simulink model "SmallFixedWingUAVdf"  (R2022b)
settings: Solver=ode4  StartTime=0  StopTime=stoptime  FixedStep=0.001  RelTol=1e-3  EnableMultiTasking=on
PreLoadFcn:
  | asbswarm_vehicledata; % load in workspace variables
PostLoadFcn:
  | open_system([gcs,'/MATLAB Animation Display/MATLAB',10,'Animation']);
InitFcn:
  | InitDatactrl
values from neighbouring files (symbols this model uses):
  env = struct    [InitDatactrl.m]
  F = Fattr + Frep    [APF.m]
  q = ix-1    [bspline_deboor.m]
  SenorSampleTime = 0.01    [InitDatactrl.m]
  sensors = struct    [InitDatactrl.m]
  uav = struct    [InitDatactrl.m]    (also in InitDatactrldf.m)
undefined symbols (not defined in the file or in its folder): Busy, Continuous, DiscIntNeverNeededParam, Dryden, Earth, Light, MIL, Newton, pa28, r, Raphson, sigbuilder_block, Wait, WGS84
libraries: simulink x37, aerolibactuator x10, sharedtransform x6, aerolibatmos2 x4, aerolibasang x4, aerolibwind2 x4, aerolibtransform2 x3, aerolibconvert2 x3, aerolibfltsims x2, shared6dof x2, aerolibnav x2, aerolibanimutils x1
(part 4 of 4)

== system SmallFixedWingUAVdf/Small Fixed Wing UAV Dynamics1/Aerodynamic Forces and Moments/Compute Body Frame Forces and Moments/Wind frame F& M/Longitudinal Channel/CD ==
  CL : Inport
  dE : Inport  Port=2
  dR : Inport  Port=3
  Apolar : Constant  Value=uav.aero.CLmin
  Apolar (A2) : Constant  Value=uav.aero.e
  Apolar (A2)1 : Constant  Value=uav.geometry.AR
  CD0 : Constant  Value=uav.aero.CD0
  CD1 : Constant  Value=uav.aero.CDDe
  CD2 : Constant  Value=uav.aero.CDDr
  Constant : Constant  Value=pi
  Product : Product  Inputs=*/  SaturateOnIntegerOverflow=on
  Product1 : Product  Inputs=***  SaturateOnIntegerOverflow=on
  Product2 : Product  SaturateOnIntegerOverflow=on
  Product4 : Product  SaturateOnIntegerOverflow=on
  Sum1 : Sum  Inputs=++++  SaturateOnIntegerOverflow=on
  Sum2 : Sum  Inputs=|+-  SaturateOnIntegerOverflow=on
  CD : Outport  VectorParamsAs1DForOutWhenUnconnected=off
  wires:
  Sum1/1 -> CD/1
  CL/1 -> Sum2/1
  CD0/1 -> Sum1/1
  Apolar/1 -> Sum2/2
  CD1/1 -> Product4/1
  dE/1 -> Product4/2
  dR/1 -> Product2/2
  CD2/1 -> Product2/1
  Sum2/1 -> Product/1
  Product4/1 -> Sum1/2
  Product2/1 -> Sum1/3
  Product/1 -> Sum1/4
  Apolar (A2)1/1 -> Product1/1
  Apolar (A2)/1 -> Product1/3
  Constant/1 -> Product1/2
  Product1/1 -> Product/2

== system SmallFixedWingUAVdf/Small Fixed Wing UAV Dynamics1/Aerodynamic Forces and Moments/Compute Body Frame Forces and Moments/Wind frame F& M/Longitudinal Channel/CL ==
  alpha : Inport
  alpha_dot : Inport  Port=2
  dE : Inport  Port=3
  dF : Inport  Port=4
  p,q,r : Inport  Port=5
  Airspeed : Inport  Port=6
  CL0 : Constant  Value=uav.aero.CL0
  CLDe : Constant  Value=uav.aero.CLDe
  CLa : Constant  Value=uav.aero.CLa
  CmDe1 : Constant  Value=uav.aero.CLDf
  Lift due to attack rate : Subsystem
  Lift due to pitch rate : Subsystem
  Product1 : Product  SaturateOnIntegerOverflow=on
  Product2 : Product  SaturateOnIntegerOverflow=on
  Product4 : Product  SaturateOnIntegerOverflow=on
  Sum : Sum  Inputs=++++++  SaturateOnIntegerOverflow=on
  CL : Outport  VectorParamsAs1DForOutWhenUnconnected=off
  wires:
  CL0/1 -> Sum/1
  Airspeed/1 -> Lift due to attack rate/1(Airspeed), Lift due to pitch rate/2(Airspeed)
  p,q,r/1 -> Lift due to pitch rate/1(p,q,r)
  Lift due to pitch rate/1(CLq) -> Sum/5
  Product2/1 -> Sum/4
  Product1/1 -> Sum/3
  CmDe1/1 -> Product2/1
  dF/1 -> Product2/2
  Sum/1 -> CL/1
  dE/1 -> Product1/2
  CLDe/1 -> Product1/1
  alpha/1 -> Product4/2
  CLa/1 -> Product4/1
  alpha_dot/1 -> Lift due to attack rate/2(alpha_dot)
  Lift due to attack rate/1(CLadot) -> Sum/6
  Product4/1 -> Sum/2

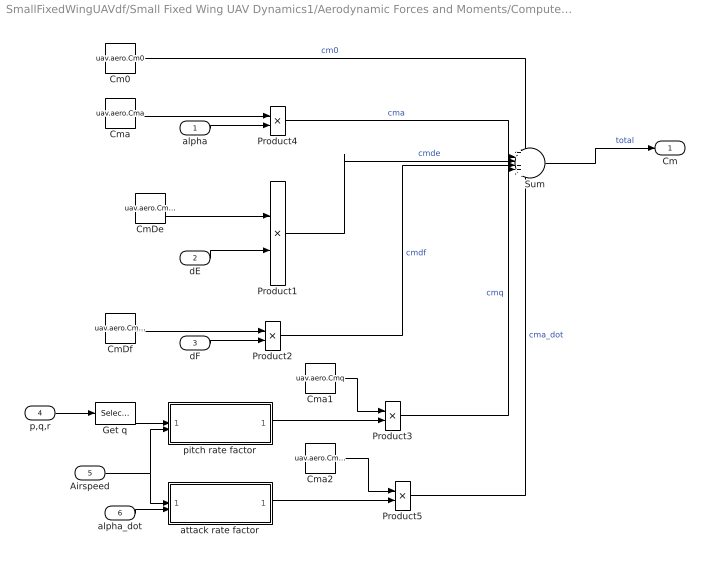
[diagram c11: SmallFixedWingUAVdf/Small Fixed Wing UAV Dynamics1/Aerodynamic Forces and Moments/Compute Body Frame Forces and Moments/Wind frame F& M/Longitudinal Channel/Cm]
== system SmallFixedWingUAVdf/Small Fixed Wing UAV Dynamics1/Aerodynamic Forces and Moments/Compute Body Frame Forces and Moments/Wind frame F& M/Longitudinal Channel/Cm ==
  alpha : Inport
  dE : Inport  Port=2
  dF : Inport  Port=3
  p,q,r : Inport  Port=4
  Airspeed : Inport  Port=5
  alpha_dot : Inport  Port=6
  Cm0 : Constant  Value=uav.aero.Cm0
  CmDe : Constant  Value=uav.aero.CmDe
  CmDf : Constant  Value=uav.aero.CmDf
  Cma : Constant  Value=uav.aero.Cma
  Cma1 : Constant  Value=uav.aero.Cmq
  Cma2 : Constant  Value=uav.aero.Cma_dot
  Get q : Selector  InputPortWidth=3  IndexOptions=Index vector (dialog)  Indices=2  OutputSizes=[(-2)]
  Product1 : Product  Inputs=**  SaturateOnIntegerOverflow=on
  Product{2..5} (4 alike) : Product  SaturateOnIntegerOverflow=on
  Sum : Sum  Inputs=++++++  SaturateOnIntegerOverflow=on
  attack rate factor : Subsystem
  pitch rate factor : Subsystem
  Cm : Outport  VectorParamsAs1DForOutWhenUnconnected=off
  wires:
  Product3/1 -> Sum/5  "cmq"
  p,q,r/1 -> Get q/1
  Product1/1 -> Sum/3  "cmde"
  Product4/1 -> Sum/2  "cma"
  Sum/1 -> Cm/1  "total"
  dE/1 -> Product1/2
  CmDe/1 -> Product1/1
  alpha/1 -> Product4/2
  Cma/1 -> Product4/1
  dF/1 -> Product2/2
  CmDf/1 -> Product2/1
  Product2/1 -> Sum/4  "cmdf"
  Cm0/1 -> Sum/1  "cm0"
  alpha_dot/1 -> attack rate factor/2(alpha_dot)
  Get q/1 -> pitch rate factor/1(q)
  Airspeed/1 -> attack rate factor/1(Airspeed), pitch rate factor/2(Airspeed)
  Cma1/1 -> Product3/1
  pitch rate factor/1(Pitch Rate Fac) -> Product3/2
  attack rate factor/1(Pitch Rate Fac) -> Product5/2
  Cma2/1 -> Product5/1
  Product5/1 -> Sum/6  "cma_dot"

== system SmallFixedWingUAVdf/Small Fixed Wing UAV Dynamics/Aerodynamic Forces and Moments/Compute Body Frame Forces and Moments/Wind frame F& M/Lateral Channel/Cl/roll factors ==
  p,q,r : Inport
  Airspeed : Inport  Port=2
  Constant : Constant  Value=uav.aero.Clp
  Constant1 : Constant  Value=uav.aero.Clr
  Get p : Selector  InputPortWidth=3  IndexOptions=Index vector (dialog)  Indices=1  OutputSizes=[(-2)]
  Get r : Selector  InputPortWidth=3  IndexOptions=Index vector (dialog)  Indices=3  OutputSizes=[(-2)]
  Product : Product  SaturateOnIntegerOverflow=on
  Product1 : Product  SaturateOnIntegerOverflow=on
  roll rate fact : Subsystem
  yaw rate fact1 : Subsystem
  Clp : Outport  VectorParamsAs1DForOutWhenUnconnected=off
  Clr : Outport  Port=2  VectorParamsAs1DForOutWhenUnconnected=off
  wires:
  Get r/1 -> yaw rate fact1/1(r)
  p,q,r/1 -> Get r/1, Get p/1
  Get p/1 -> roll rate fact/1(p)
  Airspeed/1 -> yaw rate fact1/2(Airspeed), roll rate fact/2(Airspeed)
  yaw rate fact1/1(Yaw Rate Fac) -> Product1/2
  Constant1/1 -> Product1/1
  roll rate fact/1(Roll Rate Fac) -> Product/2
  Constant/1 -> Product/1
  Product1/1 -> Clr/1
  Product/1 -> Clp/1

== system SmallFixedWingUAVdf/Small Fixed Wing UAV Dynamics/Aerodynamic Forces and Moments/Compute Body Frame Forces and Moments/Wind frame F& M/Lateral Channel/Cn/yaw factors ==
  p,q,r : Inport
  Airspeed : Inport  Port=2
  Constant : Constant  Value=uav.aero.Cnp
  Constant1 : Constant  Value=uav.aero.Cnr
  Get p : Selector  InputPortWidth=3  IndexOptions=Index vector (dialog)  Indices=1  OutputSizes=[(-2)]
  Get r : Selector  InputPortWidth=3  IndexOptions=Index vector (dialog)  Indices=3  OutputSizes=[(-2)]
  Product : Product  SaturateOnIntegerOverflow=on
  Product1 : Product  SaturateOnIntegerOverflow=on
  roll rate fact : Subsystem
  yaw rate fact : Subsystem
  Cnp : Outport  VectorParamsAs1DForOutWhenUnconnected=off
  Cnr : Outport  Port=2  VectorParamsAs1DForOutWhenUnconnected=off
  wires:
  Airspeed/1 -> yaw rate fact/2(Airspeed), roll rate fact/2(Airspeed)
  Get r/1 -> yaw rate fact/1(r)
  p,q,r/1 -> Get r/1, Get p/1
  Get p/1 -> roll rate fact/1(p)
  roll rate fact/1(Roll Rate Fac) -> Product/2
  Constant/1 -> Product/1
  yaw rate fact/1(Yaw Rate Fac) -> Product1/2
  Constant1/1 -> Product1/1
  Product1/1 -> Cnr/1
  Product/1 -> Cnp/1

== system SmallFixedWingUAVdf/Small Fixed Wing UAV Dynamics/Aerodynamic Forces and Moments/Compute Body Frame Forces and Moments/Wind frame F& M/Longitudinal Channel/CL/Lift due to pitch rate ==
  p,q,r : Inport
  Airspeed : Inport  Port=2
  Constant : Constant  Value=uav.aero.CLq
  Get q : Selector  InputPortWidth=3  IndexOptions=Index vector (dialog)  Indices=2  OutputSizes=[(-2)]
  Product : Product  SaturateOnIntegerOverflow=on
  pitch rate factor : Subsystem
  CLq : Outport  VectorParamsAs1DForOutWhenUnconnected=off
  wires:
  Airspeed/1 -> pitch rate factor/2(Airspeed)
  Get q/1 -> pitch rate factor/1(q)
  p,q,r/1 -> Get q/1
  Product/1 -> CLq/1
  pitch rate factor/1(Pitch Rate Fac) -> Product/2
  Constant/1 -> Product/1

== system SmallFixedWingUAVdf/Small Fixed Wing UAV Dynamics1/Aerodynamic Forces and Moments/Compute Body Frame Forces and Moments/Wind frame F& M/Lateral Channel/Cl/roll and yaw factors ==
  p,q,r : Inport
  Airspeed : Inport  Port=2
  Constant : Constant  Value=uav.aero.Clp
  Constant1 : Constant  Value=uav.aero.Clr
  Get p : Selector  InputPortWidth=3  IndexOptions=Index vector (dialog)  Indices=1  OutputSizes=[(-2)]
  Get r : Selector  InputPortWidth=3  IndexOptions=Index vector (dialog)  Indices=3  OutputSizes=[(-2)]
  Product : Product  SaturateOnIntegerOverflow=on
  Product1 : Product  SaturateOnIntegerOverflow=on
  roll rate fact : Subsystem
  yaw rate fact : Subsystem
  Clp : Outport  VectorParamsAs1DForOutWhenUnconnected=off
  Clr : Outport  Port=2  VectorParamsAs1DForOutWhenUnconnected=off
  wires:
  Get r/1 -> yaw rate fact/1(r)
  p,q,r/1 -> Get r/1, Get p/1
  Get p/1 -> roll rate fact/1(p)
  Airspeed/1 -> yaw rate fact/2(Airspeed), roll rate fact/2(Airspeed)
  yaw rate fact/1(Yaw Rate Fac) -> Product1/2
  Constant1/1 -> Product1/1
  roll rate fact/1(Roll Rate Fac) -> Product/2
  Constant/1 -> Product/1
  Product1/1 -> Clr/1
  Product/1 -> Clp/1

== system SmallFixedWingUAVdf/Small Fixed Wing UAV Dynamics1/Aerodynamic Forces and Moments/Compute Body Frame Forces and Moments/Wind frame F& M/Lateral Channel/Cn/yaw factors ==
  p,q,r : Inport
  Airspeed : Inport  Port=2
  Constant : Constant  Value=uav.aero.Cnp
  Constant1 : Constant  Value=uav.aero.Cnr
  Get p : Selector  InputPortWidth=3  IndexOptions=Index vector (dialog)  Indices=1  OutputSizes=[(-2)]
  Get r : Selector  InputPortWidth=3  IndexOptions=Index vector (dialog)  Indices=3  OutputSizes=[(-2)]
  Product : Product  SaturateOnIntegerOverflow=on
  Product1 : Product  SaturateOnIntegerOverflow=on
  roll rate fact : Subsystem
  yaw rate fact : Subsystem
  Cnp : Outport  VectorParamsAs1DForOutWhenUnconnected=off
  Cnr : Outport  Port=2  VectorParamsAs1DForOutWhenUnconnected=off
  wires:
  Airspeed/1 -> yaw rate fact/2(Airspeed), roll rate fact/2(Airspeed)
  Get r/1 -> yaw rate fact/1(r)
  p,q,r/1 -> Get r/1, Get p/1
  Get p/1 -> roll rate fact/1(p)
  roll rate fact/1(Roll Rate Fac) -> Product/2
  Constant/1 -> Product/1
  yaw rate fact/1(Yaw Rate Fac) -> Product1/2
  Constant1/1 -> Product1/1
  Product1/1 -> Cnr/1
  Product/1 -> Cnp/1

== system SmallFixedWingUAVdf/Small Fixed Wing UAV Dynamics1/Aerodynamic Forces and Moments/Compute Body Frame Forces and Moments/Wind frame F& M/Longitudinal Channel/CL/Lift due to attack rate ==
  Airspeed : Inport
  alpha_dot : Inport  Port=2
  CLa_dot : Constant  Value=uav.aero.CLa_dot
  Product : Product  SaturateOnIntegerOverflow=on
  attack rate factor : Subsystem
  CLadot : Outport  VectorParamsAs1DForOutWhenUnconnected=off
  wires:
  Airspeed/1 -> attack rate factor/1(Airspeed)
  alpha_dot/1 -> attack rate factor/2(alpha_dot)
  Product/1 -> CLadot/1
  attack rate factor/1(Pitch Rate Fac) -> Product/2
  CLa_dot/1 -> Product/1

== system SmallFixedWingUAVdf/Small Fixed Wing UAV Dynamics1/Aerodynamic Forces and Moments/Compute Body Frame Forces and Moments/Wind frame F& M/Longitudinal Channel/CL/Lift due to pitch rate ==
  p,q,r : Inport
  Airspeed : Inport  Port=2
  Constant : Constant  Value=uav.aero.CLq
  Get q : Selector  InputPortWidth=3  IndexOptions=Index vector (dialog)  Indices=2  OutputSizes=[(-2)]
  Product : Product  SaturateOnIntegerOverflow=on
  pitch rate factor : Subsystem
  CLq : Outport  VectorParamsAs1DForOutWhenUnconnected=off
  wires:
  Airspeed/1 -> pitch rate factor/2(Airspeed)
  Get q/1 -> pitch rate factor/1(q)
  p,q,r/1 -> Get q/1
  Product/1 -> CLq/1
  pitch rate factor/1(Pitch Rate Fac) -> Product/2
  Constant/1 -> Product/1

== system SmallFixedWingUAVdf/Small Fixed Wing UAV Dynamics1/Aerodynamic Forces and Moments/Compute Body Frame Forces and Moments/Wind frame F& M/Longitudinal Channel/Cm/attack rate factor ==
  Airspeed : Inport
  alpha_dot : Inport  Port=2
  Cmq2 : Constant  Value=uav.geometry.chord
  Cmq3 : Constant  Value=.5
  Product : Product  Inputs=***/  SaturateOnIntegerOverflow=on
  Saturation : Saturate  UpperLimit=inf  LowerLimit=0.1
  Pitch Rate Fac : Outport  VectorParamsAs1DForOutWhenUnconnected=off
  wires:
  Saturation/1 -> Product/4
  Cmq2/1 -> Product/2
  Airspeed/1 -> Saturation/1
  Product/1 -> Pitch Rate Fac/1
  alpha_dot/1 -> Product/1
  Cmq3/1 -> Product/3

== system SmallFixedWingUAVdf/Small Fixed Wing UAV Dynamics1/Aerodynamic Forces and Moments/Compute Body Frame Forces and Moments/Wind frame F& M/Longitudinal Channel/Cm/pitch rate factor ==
  q : Inport
  Airspeed : Inport  Port=2
  Cmq2 : Constant  Value=uav.geometry.chord
  Cmq3 : Constant  Value=.5
  Product : Product  Inputs=***/  SaturateOnIntegerOverflow=on
  Saturation : Saturate  UpperLimit=inf  LowerLimit=0.1
  Pitch Rate Fac : Outport  VectorParamsAs1DForOutWhenUnconnected=off
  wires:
  Saturation/1 -> Product/4
  Cmq2/1 -> Product/2
  Airspeed/1 -> Saturation/1
  q/1 -> Product/1
  Product/1 -> Pitch Rate Fac/1
  Cmq3/1 -> Product/3

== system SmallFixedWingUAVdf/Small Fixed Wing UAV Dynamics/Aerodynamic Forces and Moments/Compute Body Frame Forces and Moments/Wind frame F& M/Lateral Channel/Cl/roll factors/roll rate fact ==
  p : Inport
  Airspeed : Inport  Port=2
  Cmq1 : Constant  Value=.5
  Cmq2 : Constant  Value=uav.geometry.span
  Product : Product  Inputs=***/  SaturateOnIntegerOverflow=on
  Saturation : Saturate  UpperLimit=inf  LowerLimit=0.1
  Roll Rate Fac : Outport  VectorParamsAs1DForOutWhenUnconnected=off
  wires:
  Saturation/1 -> Product/4
  Airspeed/1 -> Saturation/1
  Cmq2/1 -> Product/3
  Cmq1/1 -> Product/2
  p/1 -> Product/1
  Product/1 -> Roll Rate Fac/1

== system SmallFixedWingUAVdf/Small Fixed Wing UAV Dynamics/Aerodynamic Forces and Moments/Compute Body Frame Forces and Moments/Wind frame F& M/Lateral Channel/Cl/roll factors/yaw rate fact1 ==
  r : Inport
  Airspeed : Inport  Port=2
  Cmq3 : Constant  Value=.5
  Cmq4 : Constant  Value=uav.geometry.span
  Product1 : Product  Inputs=***/  SaturateOnIntegerOverflow=on
  Saturation : Saturate  UpperLimit=inf  LowerLimit=0.1
  Yaw Rate Fac : Outport  VectorParamsAs1DForOutWhenUnconnected=off
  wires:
  Saturation/1 -> Product1/4
  Airspeed/1 -> Saturation/1
  Cmq4/1 -> Product1/3
  Cmq3/1 -> Product1/2
  r/1 -> Product1/1
  Product1/1 -> Yaw Rate Fac/1

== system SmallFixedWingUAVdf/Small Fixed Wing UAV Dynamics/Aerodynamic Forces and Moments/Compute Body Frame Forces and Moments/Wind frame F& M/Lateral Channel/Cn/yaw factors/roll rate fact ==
  p : Inport
  Airspeed : Inport  Port=2
  Cmq1 : Constant  Value=.5
  Cmq2 : Constant  Value=uav.geometry.span
  Product : Product  Inputs=***/  SaturateOnIntegerOverflow=on
  Saturation : Saturate  UpperLimit=inf  LowerLimit=0.1
  Roll Rate Fac : Outport  VectorParamsAs1DForOutWhenUnconnected=off
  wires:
  Saturation/1 -> Product/4
  Airspeed/1 -> Saturation/1
  Cmq2/1 -> Product/3
  Cmq1/1 -> Product/2
  p/1 -> Product/1
  Product/1 -> Roll Rate Fac/1

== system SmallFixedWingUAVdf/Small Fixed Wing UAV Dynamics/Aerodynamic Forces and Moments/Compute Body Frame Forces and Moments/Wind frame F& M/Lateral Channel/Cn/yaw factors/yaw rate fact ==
  r : Inport
  Airspeed : Inport  Port=2
  Cmq3 : Constant  Value=.5
  Cmq4 : Constant  Value=uav.geometry.span
  Product1 : Product  Inputs=***/  SaturateOnIntegerOverflow=on
  Saturation : Saturate  UpperLimit=inf  LowerLimit=0.1
  Yaw Rate Fac : Outport  VectorParamsAs1DForOutWhenUnconnected=off
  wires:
  Product1/1 -> Yaw Rate Fac/1
  r/1 -> Product1/1
  Cmq3/1 -> Product1/2
  Cmq4/1 -> Product1/3
  Airspeed/1 -> Saturation/1
  Saturation/1 -> Product1/4

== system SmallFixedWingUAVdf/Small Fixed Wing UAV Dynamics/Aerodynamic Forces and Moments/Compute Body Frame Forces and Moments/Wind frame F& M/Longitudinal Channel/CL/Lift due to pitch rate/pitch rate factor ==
  q : Inport
  Airspeed : Inport  Port=2
  Cmq2 : Constant  Value=uav.geometry.chord
  Product : Product  Inputs=**/  SaturateOnIntegerOverflow=on
  Saturation : Saturate  UpperLimit=inf  LowerLimit=0.1
  Pitch Rate Fac : Outport  VectorParamsAs1DForOutWhenUnconnected=off
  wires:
  Saturation/1 -> Product/3
  Cmq2/1 -> Product/2
  Airspeed/1 -> Saturation/1
  q/1 -> Product/1
  Product/1 -> Pitch Rate Fac/1

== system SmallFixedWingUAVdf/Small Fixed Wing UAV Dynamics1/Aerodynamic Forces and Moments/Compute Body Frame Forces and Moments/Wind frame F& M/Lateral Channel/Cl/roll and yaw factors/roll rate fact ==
  p : Inport
  Airspeed : Inport  Port=2
  Cmq1 : Constant  Value=.5
  Cmq2 : Constant  Value=uav.geometry.span
  Product : Product  Inputs=***/  SaturateOnIntegerOverflow=on
  Saturation : Saturate  UpperLimit=inf  LowerLimit=0.1
  Roll Rate Fac : Outport  VectorParamsAs1DForOutWhenUnconnected=off
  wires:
  Saturation/1 -> Product/4
  Airspeed/1 -> Saturation/1
  Cmq2/1 -> Product/3
  Cmq1/1 -> Product/2
  p/1 -> Product/1
  Product/1 -> Roll Rate Fac/1

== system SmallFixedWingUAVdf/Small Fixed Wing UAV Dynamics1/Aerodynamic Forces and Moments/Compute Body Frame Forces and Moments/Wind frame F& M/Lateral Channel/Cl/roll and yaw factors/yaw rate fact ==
  r : Inport
  Airspeed : Inport  Port=2
  Cmq3 : Constant  Value=.5
  Cmq4 : Constant  Value=uav.geometry.span
  Product1 : Product  Inputs=***/  SaturateOnIntegerOverflow=on
  Saturation : Saturate  UpperLimit=inf  LowerLimit=0.1
  Yaw Rate Fac : Outport  VectorParamsAs1DForOutWhenUnconnected=off
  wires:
  Product1/1 -> Yaw Rate Fac/1
  r/1 -> Product1/1
  Cmq3/1 -> Product1/2
  Cmq4/1 -> Product1/3
  Airspeed/1 -> Saturation/1
  Saturation/1 -> Product1/4

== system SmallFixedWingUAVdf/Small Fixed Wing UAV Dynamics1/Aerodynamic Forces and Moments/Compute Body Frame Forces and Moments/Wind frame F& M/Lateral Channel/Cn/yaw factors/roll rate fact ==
  p : Inport
  Airspeed : Inport  Port=2
  Cmq1 : Constant  Value=.5
  Cmq2 : Constant  Value=uav.geometry.span
  Product : Product  Inputs=***/  SaturateOnIntegerOverflow=on
  Saturation : Saturate  UpperLimit=inf  LowerLimit=0.1
  Roll Rate Fac : Outport  VectorParamsAs1DForOutWhenUnconnected=off
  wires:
  Saturation/1 -> Product/4
  Airspeed/1 -> Saturation/1
  Cmq2/1 -> Product/3
  Cmq1/1 -> Product/2
  p/1 -> Product/1
  Product/1 -> Roll Rate Fac/1

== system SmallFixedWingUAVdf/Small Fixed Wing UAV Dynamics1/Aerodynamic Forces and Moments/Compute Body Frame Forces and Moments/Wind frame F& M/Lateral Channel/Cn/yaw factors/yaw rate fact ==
  r : Inport
  Airspeed : Inport  Port=2
  Cmq3 : Constant  Value=.5
  Cmq4 : Constant  Value=uav.geometry.span
  Product1 : Product  Inputs=***/  SaturateOnIntegerOverflow=on
  Saturation : Saturate  UpperLimit=inf  LowerLimit=0.1
  Yaw Rate Fac : Outport  VectorParamsAs1DForOutWhenUnconnected=off
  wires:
  Product1/1 -> Yaw Rate Fac/1
  r/1 -> Product1/1
  Cmq3/1 -> Product1/2
  Cmq4/1 -> Product1/3
  Airspeed/1 -> Saturation/1
  Saturation/1 -> Product1/4

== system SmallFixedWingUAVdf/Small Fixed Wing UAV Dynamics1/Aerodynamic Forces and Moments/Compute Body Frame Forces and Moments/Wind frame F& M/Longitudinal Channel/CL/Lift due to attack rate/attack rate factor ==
  Airspeed : Inport
  alpha_dot : Inport  Port=2
  Cmq2 : Constant  Value=uav.geometry.chord
  Product : Product  Inputs=**/  SaturateOnIntegerOverflow=on
  Saturation : Saturate  UpperLimit=inf  LowerLimit=0.1
  Pitch Rate Fac : Outport  VectorParamsAs1DForOutWhenUnconnected=off
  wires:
  Saturation/1 -> Product/3
  Cmq2/1 -> Product/2
  Airspeed/1 -> Saturation/1
  Product/1 -> Pitch Rate Fac/1
  alpha_dot/1 -> Product/1

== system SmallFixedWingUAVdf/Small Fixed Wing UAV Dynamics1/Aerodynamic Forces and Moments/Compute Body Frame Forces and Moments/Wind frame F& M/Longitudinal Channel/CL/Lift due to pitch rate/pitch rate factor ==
  q : Inport
  Airspeed : Inport  Port=2
  Cmq2 : Constant  Value=uav.geometry.chord
  Product : Product  Inputs=**/  SaturateOnIntegerOverflow=on
  Saturation : Saturate  UpperLimit=inf  LowerLimit=0.1
  Pitch Rate Fac : Outport  VectorParamsAs1DForOutWhenUnconnected=off
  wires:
  Saturation/1 -> Product/3
  Cmq2/1 -> Product/2
  Airspeed/1 -> Saturation/1
  q/1 -> Product/1
  Product/1 -> Pitch Rate Fac/1

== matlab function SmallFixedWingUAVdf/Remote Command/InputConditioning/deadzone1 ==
function y = fcn(u)
%Function description:
%  Control the range of the remote control input from RCMin to RCMax, and set
%  a dead zone with a dead zone size of ±deadZone,the output y is
%  normalized to 0~1.You can get the RC calibration parameters in QGC.
RCMin = 1100;
RCMax = 1900;
RCMid = (RCMin + RCMax)/2;
deadZoneRate = 0.05;
deadZone = deadZoneRate*(RCMax - RCMin);
k = 1/(RCMax - RCMid - deadZone);
%Limiting
if(u < RCMin)
    u = RCMin;
elseif(u > RCMax)
    u = RCMax;
end
%dead zone and normalize
 if(u > RCMid + deadZone)
    y = (u-RCMid - deadZone)*k;
 elseif(u < RCMid - deadZone)
     y = (u - RCMid + deadZone)*k;
 else
     y = 0;
 end

 end

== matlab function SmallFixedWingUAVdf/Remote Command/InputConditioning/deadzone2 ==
function y = fcn(u)
%Function description:
%  Control the range of the remote control input from RCMin to RCMax, and set
%  a dead zone with a dead zone size of ±deadZone,the output y is
%  normalized to 0~1.You can get the RC calibration parameters in QGC.
RCMin = 1100;
RCMax = 1900;
RCMid = (RCMin + RCMax)/2;
deadZoneRate = 0.05;
deadZone = deadZoneRate*(RCMax - RCMin);
k = 1/(RCMax - RCMid - deadZone);
%Limiting
if(u < RCMin)
    u = RCMin;
elseif(u > RCMax)
    u = RCMax;
end
%dead zone and normalize
 if(u > RCMid + deadZone)
    y = (u-RCMid - deadZone)*k;
 elseif(u < RCMid - deadZone)
     y = (u - RCMid + deadZone)*k;
 else
     y = 0;
 end

 end

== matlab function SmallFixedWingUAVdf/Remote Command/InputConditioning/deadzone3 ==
function y = fcn(u)
%Function description:
%  Control the range of the remote control input from RCMin to RCMax, and set
%  a dead zone with a dead zone size of ±deadZone,the output y is
%  normalized to 0~1.You can get the RC calibration parameters in QGC.
RCMin = 1100;
RCMax = 1900;
RCMid = (RCMin + RCMax)/2;
deadZoneRate = 0.05;
deadZone = deadZoneRate*(RCMax - RCMin);
k = 1/(RCMax - RCMid - deadZone);
%Limiting
if(u < RCMin)
    u = RCMin;
elseif(u > RCMax)
    u = RCMax;
end
%dead zone and normalize
 if(u > RCMid + deadZone)
    y = (u-RCMid - deadZone)*k;
 elseif(u < RCMid - deadZone)
     y = (u - RCMid + deadZone)*k;
 else
     y = 0;
 end

 end

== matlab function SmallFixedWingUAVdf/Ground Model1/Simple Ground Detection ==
function ifGround = Ground(Xe3)
if Xe3>-(1e-3)
    ifGround = 1;
else
    ifGround = 0;
end

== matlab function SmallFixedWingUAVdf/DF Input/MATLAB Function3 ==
function [av1,Hz,yaw,roll] = DF(xd,dxd,ddxd,x,dx,g)
    
%     x1 = (xd-x)/norm(xd-x);

    r1 = (dxd)/norm(dxd);
    
    av1 =  r1'*(1*ddxd-[0;0;g]+3*(dxd-dx)+0.1*(xd-x));

    an = (eye(3)-r1*r1')*(ddxd-[0;0;g]);

    av3 = -(norm(an));
    
    Hz = xd(3);

    r3 = an/av3;

    r2 = cross(r3,r1);

    yaw = atan2(r1(2),r1(1));
    
    roll = atan2(r2(3),r3(3));

    if isnan(av1)
        av1=0;
    end
    if isnan(Hz)
        Hz=0;
    end
    if isnan(yaw)
        yaw=0;
    end

end

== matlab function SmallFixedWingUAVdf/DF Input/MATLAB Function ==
function roll = fcn(yaw,yawdes,g,V,rolldes)
%     roll = yawrate*g*V;
    if yaw>pi
        yaw = yaw-2*pi;
    end
    yawrate1 = 0.7*(yawdes-yaw);
    roll = atan2(V.*(yawrate1),g);
end

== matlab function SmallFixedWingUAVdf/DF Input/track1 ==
function [Xd,Vd,Ad,Jd] = fcn(x,y,dx,dy,ddx,ddy,dddx,dddy)
    Xd = [x,-y,100]';
    Vd = [dx,-dy,0]';
    Ad = [ddx,-ddy,0]';
    Jd = [dddx,-dddy,0]';
end

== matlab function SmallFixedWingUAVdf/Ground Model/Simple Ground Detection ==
function ifGround = Ground(Xe3)
if Xe3>-(1e-3)
    ifGround = 1;
else
    ifGround = 0;
end

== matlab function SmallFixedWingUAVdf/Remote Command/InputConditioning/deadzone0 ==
function y = fcn(u)
%Function description:
%  Control the range of the remote control input from RCMin to RCMax,which can be obtained from QGC. And set
%  a dead zone with a dead zone size of deadZone,the output y is normalized to 0~1.
RCMin = 1100;
RCMax = 1900;
RCMid = (RCMin + RCMax)/2;
deadZoneRate = 0.05;
deadZone = deadZoneRate*(RCMax - RCMin);
k = 1/(RCMax - RCMid - deadZone);
%Limiting
if(u < RCMin)
    u = RCMin;
elseif(u > RCMax)
    u = RCMax;
end
%dead zone and normalize
 if(u > RCMid + deadZone)
    y = (u-RCMid - deadZone)*k;
 elseif(u < RCMid - deadZone)
     y = (u - RCMid + deadZone)*k;
 else
     y = 0;
 end

 end
